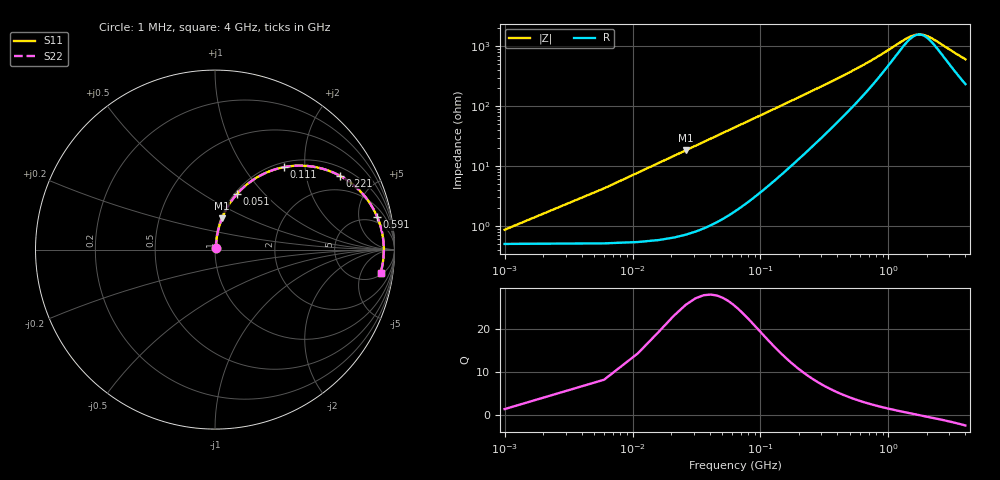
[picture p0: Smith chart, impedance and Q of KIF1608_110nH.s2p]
# MHz S RI R 50
!Freq ReS11 ImS11 ReS21 ImS21 ReS12 ImS12 ReS22 ImS22
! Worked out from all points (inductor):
!   801 points, 1 MHz to 4 GHz, reference 50 ohm
!   read as one part in series: L = 112 nH near 21 MHz
!   highest Q = 24.9 at 26 MHz (marker M1), where L = 112 nH
!   self-resonance near 1.746 GHz
!   S11 on the Smith chart (normalised r, x): 1 MHz: 1.01, +0.01; 51 MHz: 1.03, +0.72; 111 MHz: 1.09, +1.56; 221 MHz: 1.32, +3.13; 591 MHz: 3.56, +8.63; 4 GHz: 6, -11
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1  0.00503 0.00696  0.995 -0.00696  0.995 -0.00696  0.00503 0.00696
11  0.0112 0.0761  0.9888 -0.0761  0.9888 -0.0761  0.0112 0.0761
26  0.0388 0.1745  0.9612 -0.1745  0.9612 -0.1745  0.0388 0.1745
31  0.0523 0.205  0.9477 -0.205  0.9477 -0.205  0.0523 0.205
36  0.0677 0.2339  0.9323 -0.2339  0.9323 -0.2339  0.0677 0.2339
51  0.1229 0.3105  0.8771 -0.3105  0.8771 -0.3105  0.1229 0.3105
76  0.2323 0.4013  0.7677 -0.4013  0.7677 -0.4013  0.2323 0.4013
111  0.3862 0.4598  0.6138 -0.4598  0.6138 -0.4598  0.3862 0.4598
166  0.5742 0.4568  0.4258 -0.4568  0.4258 -0.4568  0.5742 0.4568
221  0.6939 0.4123  0.3061 -0.4123  0.3061 -0.4123  0.6939 0.4123
281  0.7738 0.3582  0.2262 -0.3582  0.2262 -0.3582  0.7738 0.3582
361  0.8352 0.2959  0.1648 -0.2959  0.1648 -0.2959  0.8352 0.2959
591  0.9043 0.1811  0.0957 -0.1811  0.0957 -0.1811  0.9043 0.1811
671  0.9142 0.1552  0.0858 -0.1552  0.0858 -0.1552  0.9142 0.1552
1011  0.9335 0.082  0.0665 -0.082  0.0665 -0.082  0.9335 0.082
1336  0.9391 0.0389  0.0609 -0.0389  0.0609 -0.0389  0.9391 0.0389
1501  0.9402 0.0218  0.0598 -0.0218  0.0598 -0.0218  0.9402 0.0218
1656  0.9407 0.00759  0.0593 -0.00759  0.0593 -0.00759  0.9407 0.00759
2001  0.9404 -0.0197  0.0596 0.0197  0.0596 0.0197  0.9404 -0.0197
2671  0.9365 -0.0629  0.0635 0.0629  0.0635 0.0629  0.9365 -0.0629
3336  0.9303 -0.0989  0.0697 0.0989  0.0697 0.0989  0.9303 -0.0989
4000  0.9221 -0.131  0.0779 0.131  0.0779 0.131  0.9221 -0.131
